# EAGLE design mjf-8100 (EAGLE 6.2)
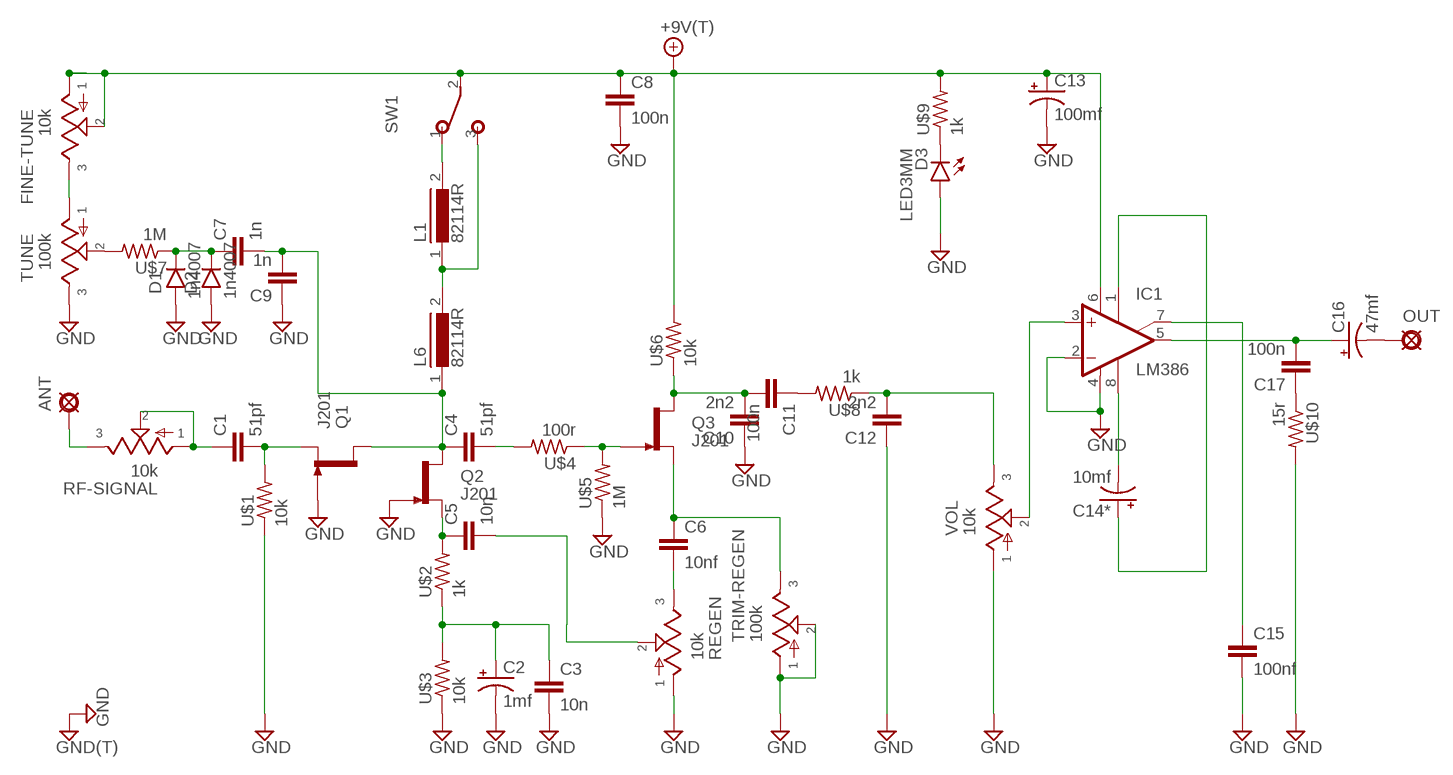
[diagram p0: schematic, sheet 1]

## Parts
+9V1  +9V(T)  [SQUARE]
ANT  PADL  [LONG]
C1  51pf  050X030_0252  [050X030_025_2]
C2  1mf  0501  [050_020_1]
C3  10n  050X030_0502  [050X030_050]
C4  51pf  050X030_0252  [050X030_025_2]
C5  10n  050X030_0252  [050X030_025_2]
C6  10nf  050X030_0252  [050X030_025_2]
C7  1n  050X030_0502  [050X030_050]
C8  100n  050X030_0502  [050X030_050]
C9  1n  050X030_0251  [050X030_025]
C10  2n2  050X030_0502  [050X030_050]
C11  100n  050X030_0502  [050X030_050]
C12  2n2  050X030_0502  [050X030_050]
C13  100mf  0501  [050_020_1]
C14*  10mf  0501  [050_020_1]
C15  100nf  050X030_0502  [050X030_050]
C16  47mf  0501  [050_020_1]
C17  100n  050X030_0502  [050X030_050]
D1  1n4007  1N400X.3  [DO41-3]
D2  1n4007  1N400X.3  [DO41-3]
D3  LED3MM  [LED3MM]
FINE-TUNE  10k  POT16MM  [16MM]
GND22  GND(T)  [SQUARE]
IC1  LM386  [DIL08]
L1  82114R  [82114R]
L6  82114R  [82114R]
OUT  PADL  [LONG]
Q1  J201  [TO92-]
Q2  J201  [TO92-]
Q3  J201  [TO92-]
REGEN  10k  POT16MM  [16MM]
RF-SIGNAL  10k  POTTRIM3/8  [B375P]
SW1  SPDTPADS  [SPDT]
TRIM-REGEN  100k  POTTRIM3/8  [B375P]
TUNE  100k  POT16MM  [16MM]
U$1  10k  3MM.2  [R0204/2]
U$2  1k  3MM.2  [R0204/2]
U$3  10k  3MM.2  [R0204/2]
U$4  100r  3MM.2  [R0204/2]
U$5  1M  3MM.2  [R0204/2]
U$6  10k  3MM.3  [R0204/3]
U$7  1M  3MM.2  [R0204/2]
U$8  1k  3MM.2  [R0204/2]
U$9  1k  3MM.2  [R0204/2]
U$10  15r  3MM.2  [R0204/2]
VOL  10k  POT16MM  [16MM]

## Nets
+9V: +9V1.1(+9V) C8.1 C13.+ FINE-TUNE.1 FINE-TUNE.2 IC1.6(V+) SW1.2(P) U$6.2 U$9.2
GND: C2.- C3.2 C8.2 C9.1 C10.1 C12.1 C13.- C15.2 D1.A D2.A D3.A GND22.1(GND) IC1.2(-IN) IC1.4(V-) Q1.1(G) Q2.1(G) REGEN.1 TRIM-REGEN.1 TRIM-REGEN.2 TUNE.3 U$1.1 U$3.1 U$5.1 U$10.2 VOL.1
N$1: C1.2 Q1.2(S) U$1.2
N$2: C5.1 Q2.2(S) U$2.2
N$3: C2.+ C3.1 U$2.1 U$3.2
N$4: C1.1 RF-SIGNAL.1 RF-SIGNAL.2
N$5: ANT.1(PAD) RF-SIGNAL.3
N$6: C4.1 C7.2 C9.2 L6.1 Q1.3(D) Q2.3(D)
N$7: C6.1 Q3.2(S) TRIM-REGEN.3
N$8: C4.2 U$4.2
N$9: Q3.1(G) U$4.1 U$5.2
N$10: C6.2 REGEN.3
N$11: C5.2 REGEN.2
N$12: FINE-TUNE.3 TUNE.1
N$13: IC1.3(+IN) VOL.2
N$14: TUNE.2 U$7.2
N$15: C7.1 D1.C D2.C U$7.1
N$16: C10.2 C11.2 Q3.3(D) U$6.1
N$17: C12.2 U$8.1 VOL.3
N$18: C11.1 U$8.2
N$19: L1.1 L6.2 SW1.3(S)
N$20: L1.2 SW1.1(O)
N$21: C17.1 U$10.1
N$22: C14*.- IC1.8(GAIN2)
N$23: C14*.+ IC1.1(GAIN1)
N$24: C15.1 IC1.7(BYPASS)
N$25: C16.+ C17.2 IC1.5(OUT)
N$26: C16.- OUT.1(PAD)
N$27: D3.K(C) U$9.1

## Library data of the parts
+9V1 = gm-supply:+9V(T): +9V Voltage Supply
ANT OUT = gm-supply:PAD: PAD
C1 C4-C6 C9 = gm-caps-ceramic:050X030_025: 47 - 120pF
C2 C13 C14* C16 = gm-caps-electro-pol:050: 0.22 - 100uF
C3 C7 C8 C10-C12 C15 C17 = gm-caps-ceramic:050X030_050: 120 - 150pF
D1 D2 = gm-diodes:1N400X: Rectifier Diodes
D3 = gm-diodes:LED
FINE-TUNE REGEN RF-SIGNAL TRIM-REGEN TUNE VOL = gm-pots:POT: Potentiometers the arrow indicates the clockwise motion of th wiper (lug 2) fully counter clockwise there is no resistance between lugs 1 and 2 fully clockwise the resistance between lugs 1 and 2 is the value of the pot
GND22 = gm-supply:GND(T): Ground
IC1 = gm-ics:LM386: LM386 - Low Voltage Audio Power Amplifier
L1 L6 = inductors:82114R: INDUCTOR
Q1-Q3 = gm-trans:J201: N-channel JFET
SW1 = gm-switches:SPDT: TOGGLE SWITCH Marquardt
U$1-U$10 = gm-resistors:3MM: 3mm Resistors

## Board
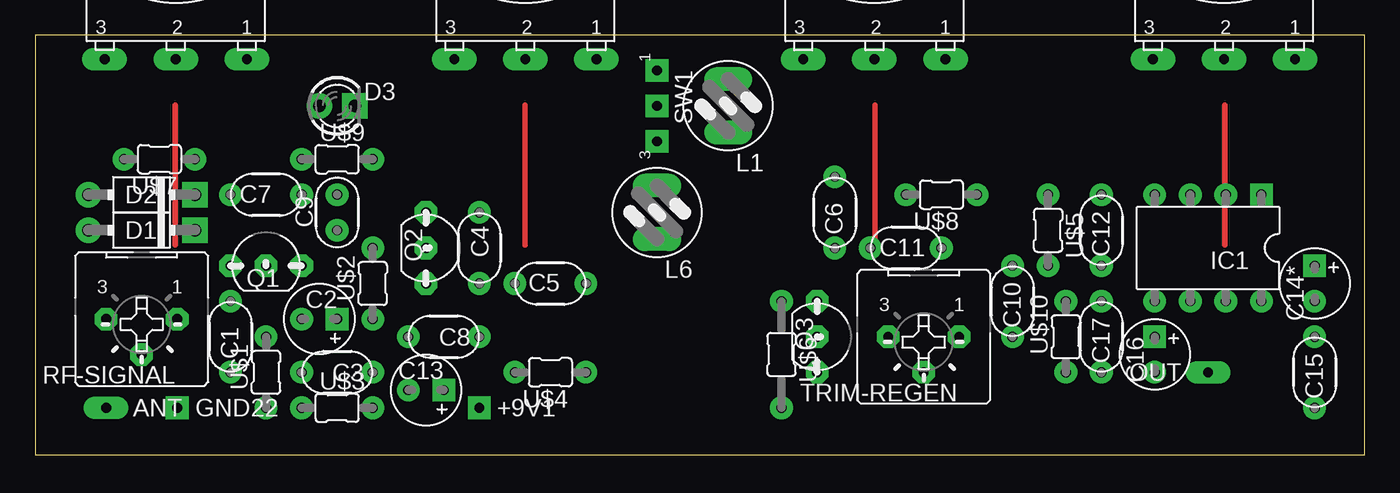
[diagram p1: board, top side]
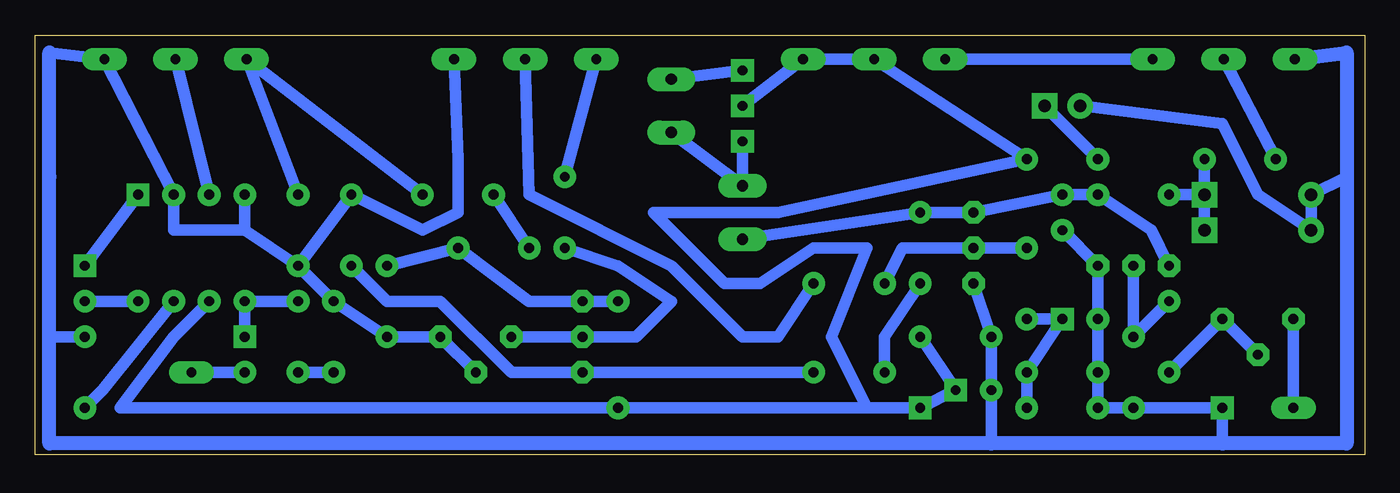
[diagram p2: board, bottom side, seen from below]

Size 95 x 30 mm. Coordinates in mm from the lower left corner, seen from the top.
Outline: 0,0 95,0 95,30 0,30 0,0
Copper layers (1*16): Top 0.035mm / dielectric 1.5mm / Bottom 0.035mm
Design rules: minimum track width 20mil, minimum drill 30mil, track to track 20mil, track to pad 20mil, pad to pad 20mil, via to via 20mil, smd to smd 8mil, copper to edge 20mil, drill to drill 10mil, minimum pad ring 18mil, minimum via ring 8mil, stop-mask expansion 4mil, vias tented up to drill 0mil, thermal gap 10mil

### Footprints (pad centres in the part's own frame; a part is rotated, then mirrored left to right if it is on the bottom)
SQUARE = drill 0.7 square: 1 0,0
LONG = drill 0.7 long: 1 0,0
050X030_025_2 = drill 0.7: 1 -2.54,0; 2 2.54,0
050_020_1 = drill 0.7 square: + -1.27,0 | drill 0.7: - 1.27,0
050X030_050 = drill 0.7: 1 -2.54,0; 2 2.54,0
050X030_025 = drill 0.7: 1 -1.27,0; 2 1.27,0
DO41-3 = drill 0.9: A 3.81,0 | drill 0.9 square: C -3.81,0
LED3MM = drill 0.9: A -1.27,0 | drill 0.9 square: K 1.27,0
16MM = drill 0.7 long: 1 5.08,0; 2 0,0; 3 -5.08,0
DIL08 = drill 0.7 square: 1 -3.81,-3.81 | drill 0.7: 2 -1.27,-3.81; 3 1.27,-3.81; 4 3.81,-3.81; 5 3.81,3.81; 6 1.27,3.81; 7 -1.27,3.81; 8 -3.81,3.81
82114R = drill 0.813 long: 1 0,1.905; 2 0,-1.905
TO92- = drill 0.7 octagon: 1 2.54,0; 2 0,0; 3 -2.54,0
B375P = drill 0.7 octagon: 1 -2.54,0; 2 0,2.54; 3 2.54,0
SPDT = drill 0.7 square: 1 -2.54,0; 2 0,0; 3 2.54,0
R0204/2 = drill 0.7: 1 -2.54,0; 2 2.54,0
R0204/3 = drill 0.7: 1 -3.81,0; 2 3.81,0

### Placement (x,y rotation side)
+9V1  31.75,3.34 0 top
ANT  5.08,3.34 0 top
C1  13.97,8.42 90 top
C2  20.32,9.69 180 top
C3  21.59,5.88 180 top
C4  31.75,14.77 270 top
C5  36.83,12.23 0 top
C6  57.15,17.31 90 top
C7  16.51,18.58 0 top
C8  29.21,8.42 180 top
C9  21.59,17.31 90 top
C10  69.85,10.96 90 top
C11  62.23,14.77 0 top
C12  76.2,16.04 90 top
C13  27.94,4.61 180 top
C14*  91.44,12.23 270 top
C15  91.44,5.88 90 top
C16  80.01,7.15 270 top
C17  76.2,8.42 90 top
D1  7.62,16.04 180 top
D2  7.62,18.58 180 top
D3  21.59,24.93 0 top
FINE-TUNE  35.04,28.27 0 top
GND22  10.16,3.34 0 top
IC1  83.82,14.77 180 top
L1  49.53,24.93 180 top
L6  44.45,17.31 180 top
OUT  83.82,5.88 180 top
Q1  16.51,13.5 0 top
Q2  27.94,14.77 270 top
Q3  55.88,8.42 270 top
REGEN  59.98,28.27 0 top
RF-SIGNAL  7.62,9.69 180 top
SW1  44.45,24.93 270 top
TRIM-REGEN  63.5,8.42 180 top
TUNE  10.06,28.27 0 top
U$1  16.51,5.88 90 top
U$2  24.13,12.23 90 top
U$3  21.59,3.34 0 top
U$4  36.83,5.88 180 top
U$5  72.39,16.04 270 top
U$6  53.34,7.15 270 top
U$7  8.89,21.12 180 top
U$8  64.77,18.58 180 top
U$9  21.59,21.12 0 top
U$10  73.66,8.42 90 top
VOL  84.96,28.27 0 top

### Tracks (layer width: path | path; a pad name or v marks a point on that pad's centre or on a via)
+9V
  Bottom 0.813: C8.1 C13.+ +9V1.1 35.56,3.34 | U$6.2 88.9,3.34 85.09,8.42 IC1.6 | U$6.2 38.1,3.34 | 38.1,3.34 36.83,3.34 | 36.83,3.34 35.56,3.34 | U$6.2 38.1,3.34 | 38.1,3.34 36.83,3.34 | SW1.2 FINE-TUNE.1 39.37,28.27 FINE-TUNE.2 U$9.2 41.91,17.31 50.8,17.31 45.72,12.23 43.18,12.23 39.37,14.77 35.56,14.77 38.1,8.42 35.56,3.34
GND
  Bottom 0.813: 1.27,19.85 D2.A D1.A 7.62,18.58 10.16,23.66 D3.A | 10.16,0.8 GND22.1 U$1.1 U$3.1 C3.2 C2.- Q1.1 C9.1 | C13.- C8.2 | TRIM-REGEN.2 TRIM-REGEN.1 C10.1 U$10.2 C12.1 | C15.2 93.98,8.42 | C8.2 26.67,0.8 | C8.2 Q2.1 | 93.98,28.74 VOL.1 IC1.2 85.09,16.04 80.01,16.04 | IC1.4 80.01,16.04 | REGEN.1 64.77,21.12 64.77,17.31 67.31,16.04 U$5.1 C12.1 | C12.1 80.01,16.04
  Bottom 1.016: 93.98,28.74 93.98,19.85 93.98,8.42 93.98,0.8 26.67,0.8 10.16,0.8 1.27,0.8 1.27,19.85 1.27,28.74 TUNE.3
N$1
  Bottom 0.813: Q1.2 U$1.2 C1.2
N$2
  Bottom 0.813: U$2.2 Q2.2 33.02,14.77 C5.1
N$3
  Bottom 0.813: U$3.2 C3.1 C2.+ U$2.1
N$4
  Bottom 0.813: RF-SIGNAL.2 RF-SIGNAL.1 C1.1
N$5
  Bottom 0.813: RF-SIGNAL.3 ANT.1
N$6
  Bottom 0.813: L6.1 C4.1 Q2.3 C9.2 C7.2 15.24,16.04 Q1.3
N$7
  Bottom 0.813: TRIM-REGEN.3 Q3.2 52.07,8.42 49.53,10.96 53.34,13.5 C6.1
N$8
  Bottom 0.813: C4.2 34.29,8.42 U$4.2
N$9
  Bottom 0.813: U$5.2 69.85,10.96 66.04,10.96 60.96,5.88 59.69,5.88 Q3.1 U$4.1
N$10
  Bottom 0.813: C6.2 REGEN.3
N$11
  Bottom 0.813: C5.2 41.91,8.42 44.45,8.42 49.53,13.5 59.69,18.58 REGEN.2
N$12
  Bottom 0.813: TUNE.1 FINE-TUNE.3
N$13
  Bottom 0.813: IC1.3 VOL.2
N$14
  Bottom 0.813: TUNE.2 U$7.2
N$15
  Bottom 0.813: D1.C D2.C | U$7.1 D2.C | D2.C C7.1
N$16
  Bottom 0.813: C10.2 C11.2 59.69,10.96 Q3.3 U$6.1
N$17
  Bottom 0.813: C12.2 VOL.3 U$8.1
N$18
  Bottom 0.813: C11.1 U$8.2
N$19
  Bottom 0.813: L1.1 L6.2 SW1.3
N$20
  Bottom 0.813: SW1.1 L1.2
N$21
  Bottom 0.813: U$10.1 C17.1
N$22
  Bottom 0.813: IC1.8 C14*.-
N$23
  Bottom 0.813: C14*.+ IC1.1
N$24
  Bottom 0.813: IC1.7 90.17,4.61 C15.1
N$25
  Bottom 0.813: C16.+ IC1.5 C17.2
N$26
  Bottom 0.813: C16.- OUT.1
N$27
  Bottom 0.813: U$9.1 D3.K
N$28
  Top 0.406: 35,25 35,15
N$29
  Top 0.406: 60,25 60,15
N$30
  Top 0.406: 85,25 85,15
N$31
  Top 0.406: 10,25 10,15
